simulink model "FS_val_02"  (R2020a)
settings: Solver=ode45  StartTime=0.0  StopTime=1000  RelTol=1e-3  EnableMultiTasking=on
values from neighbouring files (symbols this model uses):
  Ts = 0.05    [init_model.m]
libraries: fuzblock x1

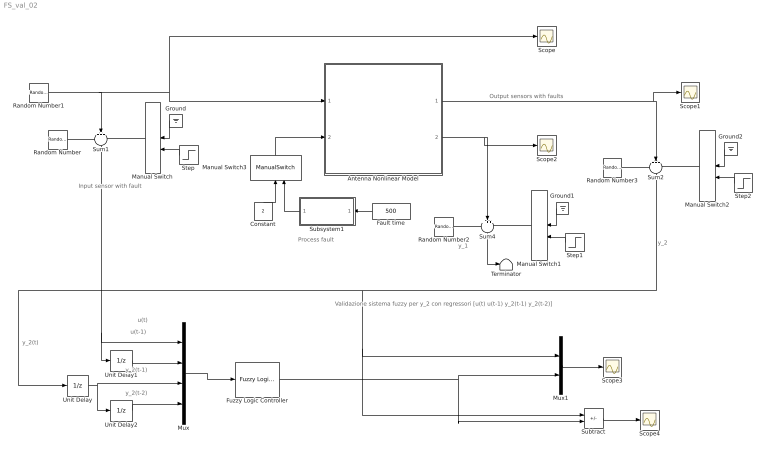
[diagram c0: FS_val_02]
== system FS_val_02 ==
  note: Validazione sistema fuzzy per y_2 con regressori [u(t) u(t-1) y_2(t-1) y_2(t-2)]
  note: y_2(t)
  note: y_2(t-1)
  note: y_1
  note: u(t)
  note: Output sensors with faults
  note: Process fault
  note: Input sensor with fault
  note: u(t-1)
  note: y_2(t-2)
  note: y_2
  Antenna Nonlinear Model : Subsystem
  Constant : Constant  Value=2
  Fault time : Constant  Value=500
  Fuzzy Logic Controller : fuzblock/Fuzzy Logic  Controller  FIS=FIS02  OutputSampleNumber=101  DataType=double  FuzzifiedInputs=off  RuleFiringStrengths=off  RuleOutputs=off  AggregatedOutputs=off  SimulateUsing=Interpreted execution  OutOfRangeInputValueMessage=warning  NoRuleFiredMessage=warning  EmptyOutputFuzzySetMessage=warning
  Ground : Ground
  Ground1 : Ground
  Ground2 : Ground
  Manual Switch{,1..3} (4 alike) : ManualSwitch
  Mux : Mux
  Mux1 : Mux  Inputs=2
  Random Number : RandomNumber  Variance=0.0001  Seed=1  SampleTime=Ts
  Random Number1 : RandomNumber  Variance=0.1  SampleTime=10
  Random Number2 : RandomNumber  Variance=0.00001  Seed=2  SampleTime=Ts
  Random Number3 : RandomNumber  Variance=0.00001  Seed=3  SampleTime=Ts
  Scope{,1..4} (5 alike) : Scope
  Step : Step  Time=500  SampleTime=0
  Step1 : Step  Time=500  SampleTime=0
  Step2 : Step  Time=500  SampleTime=0
  Subsystem1 : Subsystem
  Subtract : Sum  Inputs=+-
  Sum1 : Sum  Inputs=+++  SaturateOnIntegerOverflow=on
  Sum2 : Sum  Inputs=+++  SaturateOnIntegerOverflow=on
  Sum4 : Sum  Inputs=+++  SaturateOnIntegerOverflow=on
  Terminator : Terminator
  Unit Delay : UnitDelay  SampleTime=Ts  HasFrameUpgradeWarning=on
  Unit Delay1 : UnitDelay  SampleTime=Ts  HasFrameUpgradeWarning=on
  Unit Delay2 : UnitDelay  SampleTime=Ts  HasFrameUpgradeWarning=on
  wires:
  Random Number1/1 -> Scope/1, Antenna Nonlinear Model/1(force), Sum1/2
  Random Number/1 -> Sum1/1
  Manual Switch/1 -> Sum1/3
  Sum1/1 -> Unit Delay1/1, Mux/1
  Ground/1 -> Manual Switch/1
  Step/1 -> Manual Switch/2
  Random Number2/1 -> Sum4/1
  Ground1/1 -> Manual Switch1/1
  Manual Switch1/1 -> Sum4/3
  Step1/1 -> Manual Switch1/2
  Antenna Nonlinear Model/2(velocity) -> Sum4/2, Scope2/1
  Random Number3/1 -> Sum2/1
  Ground2/1 -> Manual Switch2/1
  Manual Switch2/1 -> Sum2/3
  Step2/1 -> Manual Switch2/2
  Antenna Nonlinear Model/1(angle) -> Sum2/2, Scope1/1
  Sum2/1 -> Subtract/1, Mux1/1, Unit Delay/1
  Fault time/1 -> Subsystem1/1(Fault time)
  Subsystem1/1(Fault) -> Manual Switch3/2
  Manual Switch3/1 -> Antenna Nonlinear Model/2(drag)
  Constant/1 -> Manual Switch3/1
  Mux/1 -> Fuzzy Logic Controller/1
  Unit Delay1/1 -> Mux/2
  Unit Delay/1 -> Unit Delay2/1, Mux/3
  Unit Delay2/1 -> Mux/4
  Mux1/1 -> Scope3/1
  Fuzzy Logic Controller/1 -> Subtract/2, Mux1/2
  Subtract/1 -> Scope4/1
  Sum4/1 -> Terminator/1

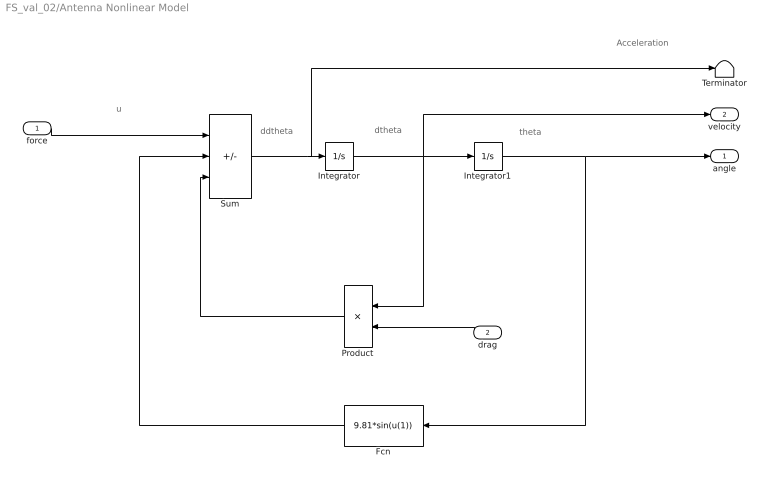
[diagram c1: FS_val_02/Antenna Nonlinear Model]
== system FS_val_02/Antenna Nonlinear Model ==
  note: Acceleration
  note: ddtheta
  note: dtheta
  note: theta
  note: u
  force : Inport
  drag : Inport  Port=2
  Fcn : Fcn  Expr=9.81*sin(u(1))
  Integrator : Integrator
  Integrator1 : Integrator  InitialCondition=(pi/180)*90
  Product : Product
  Sum : Sum  Inputs=+--  SaturateOnIntegerOverflow=on
  Terminator : Terminator
  angle : Outport
  velocity : Outport  Port=2
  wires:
  Sum/1 -> Terminator/1, Integrator/1
  Integrator/1 -> Product/1, Integrator1/1, velocity/1
  Integrator1/1 -> angle/1, Fcn/1
  Fcn/1 -> Sum/2
  Product/1 -> Sum/3
  force/1 -> Sum/1
  drag/1 -> Product/2

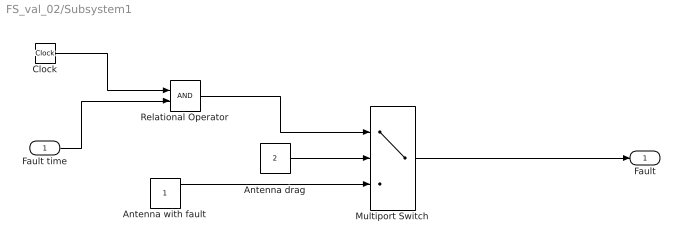
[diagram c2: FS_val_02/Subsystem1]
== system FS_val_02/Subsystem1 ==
  Fault time : Inport
  Antenna drag : Constant  Value=2
  Antenna with fault : Constant
  Clock : Clock
  Multiport Switch : MultiPortSwitch  DataPortOrder=Zero-based contiguous  Inputs=2  zeroidx=on
  Relational Operator : RelationalOperator  OutDataTypeStr=boolean  RndMeth=Simplest
  Fault : Outport
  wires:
  Clock/1 -> Relational Operator/1
  Fault time/1 -> Relational Operator/2
  Antenna drag/1 -> Multiport Switch/2
  Relational Operator/1 -> Multiport Switch/1
  Multiport Switch/1 -> Fault/1
  Antenna with fault/1 -> Multiport Switch/3
